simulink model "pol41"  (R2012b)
settings: Solver=ode45  StartTime=0.0  StopTime=10.0  RelTol=1e-3
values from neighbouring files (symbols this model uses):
  A = [0 1 0 0 0 0    [beobachter_1.m]    (also in beobachter_2.m; beobachter_22.m; kalman_1.m = my_sys.a; kalman_10.m = my_sys.a)
  B = [0 1 0 0 0 0]'    [beobachter_1.m]    (also in beobachter_2.m; beobachter_22.m; kalman_1.m = my_sys.b; kalman_10.m = my_sys.b)
  C = [0 0 0 0 1 0]    [beobachter_1.m]    (also in beobachter_2.m; beobachter_22.m; kalman_1.m = my_sys.c; kalman_10.m = my_sys.c)
  D = 0    [aktiv_tilger_1.m]    (also in aktiv_tilger_12.m; aktiv_tilger_3.m = 2000; aktiv_tilger_31.m; beobachter_1.m)
  K = Kn(1:n)    [beobachter_2.m]    (also in beobachter_22.m; LQG_1.m = lqry(sys,10,1); LQR_1.m = Kn(1:6),      ki = -Kn(7),; pol_4.m)
  ki = -Kn(n+1)    [beobachter_2.m]    (also in beobachter_22.m; kalman_12.m = -Kn(3); kalman_13.m = -Kn(4); kalman_d1.m = -Kn(4))
  Kr = 2000    [aktiv_tilger_2.m]    (also in beobachter_22.m = 5; fuellstnd_3.m = 10,; fuellstnd_31.m = 10,; kalman_12.m = Kn(1:2))
  smax = 0.05    [beobachter_22.m]    (also in PID_windup1.m = 0.3; pol_41.m = 0.02)

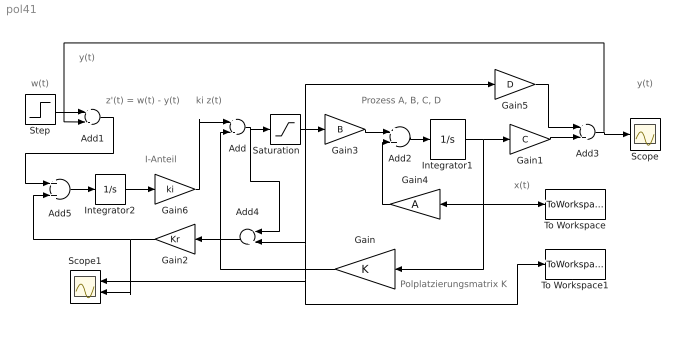
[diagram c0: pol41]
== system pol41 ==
  note: z'(t) = w(t) - y(t)
  note: y(t)
  note: w(t)
  note: ki z(t)
  note: y(t)
  note: x(t)
  note: I-Anteil
  note: Polplatzierungsmatrix K
  note: Prozess A, B, C, D
  Add : Sum  Inputs=+-
  Add1 : Sum  Inputs=+-
  Add2 : Sum
  Add3 : Sum
  Add4 : Sum  Inputs=-+
  Add5 : Sum
  Gain : Gain  Gain=K  Multiplication=Matrix(K*u)
  Gain1 : Gain  Gain=C  Multiplication=Matrix(K*u)
  Gain2 : Gain  Gain=Kr
  Gain3 : Gain  Gain=B  Multiplication=Matrix(K*u)
  Gain4 : Gain  Gain=A  Multiplication=Matrix(K*u)
  Gain5 : Gain  Gain=D  Multiplication=Matrix(K*u)
  Gain6 : Gain  Gain=ki
  Integrator1 : Integrator
  Integrator2 : Integrator
  Saturation : Saturate  UpperLimit=smax  LowerLimit=-smax  LinearizeAsGain=off  ZeroCross=off
  Scope : Scope
  Scope1 : Scope  NumInputPorts=2
  Step : Step  SampleTime=0
  To Workspace : ToWorkspace  VariableName=x  SampleTime=-1  SaveFormat=Structure With Time
  To Workspace1 : ToWorkspace  VariableName=u  SampleTime=-1  SaveFormat=Structure With Time
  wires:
  Integrator1/1 -> Gain1/1, To Workspace/1, Gain/1, Gain4/1
  Gain/1 -> Add/2
  Step/1 -> Add1/1
  Gain1/1 -> Add3/2
  Gain6/1 -> Add/1
  Add2/1 -> Integrator1/1
  Gain3/1 -> Add2/1
  Gain4/1 -> Add2/2
  Add3/1 -> Add1/2, Scope/1
  Add/1 -> Add4/1, Saturation/1
  Gain5/1 -> Add3/1
  Integrator2/1 -> Gain6/1
  Add5/1 -> Integrator2/1
  Add4/1 -> Gain2/1
  Add1/1 -> Add5/1
  Gain2/1 -> Scope1/2, Add5/2
  Saturation/1 -> To Workspace1/1, Scope1/1, Add4/2, Gain5/1, Gain3/1
